VAR_GLOBAL
	ipCreator: I_AcsiCodeCreatorClass := GVL_AcsiVars.Creator.SetCodeRev(codeRev:=3).SetGuiVer(major:=1, minor:=1, build:=94, revision:=4);
	fbIED: FB_IED_IED;
	
	fbIEDGse: FB_IEDGse := (fbAdapter:=(ipIED:=fbIED, settings:=(sMulticastAddr:='01-0C-CD-01-00-01', eDispatchMode:=E_GseDispatchMode.NonPromiscuous)));
END_VAR
